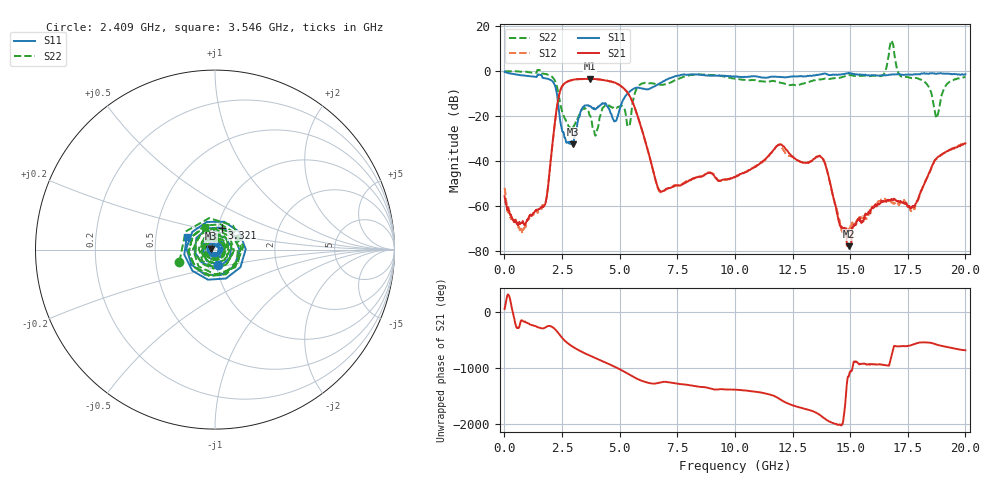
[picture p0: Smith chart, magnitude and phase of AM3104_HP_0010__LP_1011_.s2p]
!Created with skrf (http://scikit-rf.org).
# Hz S RI R 50.0
!freq ReS11 ImS11 ReS21 ImS21 ReS12 ImS12 ReS22 ImS22
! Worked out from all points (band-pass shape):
!   1601 points, 10 MHz to 20 GHz, reference 50 ohm
!   highest |S21| = -3.39 dB at 3.708 GHz (marker M1); lowest = -77.8 dB at 14.95 GHz (marker M2)
!   |S21| within 3 dB of the highest: 2.526 GHz to 5.028 GHz (2.502 GHz wide, 66.3 % of centre)
!   lowest |S11| = -32.5 dB at 2.984 GHz (marker M3), VSWR 1.05, Z = 47.7 + j0.478 ohm
!   |S11| at or under -10 dB: 2.276 GHz to 5.339 GHz (3.063 GHz wide, 80.4 % of centre)
!   |S22| runs from -28.7 to 13.6 dB; largest |S21 - S12| = 0.055
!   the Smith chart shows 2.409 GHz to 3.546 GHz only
!   S11 on the Smith chart (normalised r, x): 2.409 GHz: 1.02, -0.18; 3.321 GHz: 1.05, +0.26; 3.546 GHz: 0.72, +0.11
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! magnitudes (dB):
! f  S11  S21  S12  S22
! 10 MHz  -0.3  -55.6  -51.9  -0.1
! 722.1 MHz  -1.9  -67.5  -70.1  -0.3
! 1.697 GHz  -3.1  -60.4  -59.7  -1.1
! 2.409 GHz  -21.1  -9.1  -9.2  -13.6
! 2.984 GHz  -32.5  -3.8  -3.8  -24.8
! 3.321 GHz  -17.8  -3.5  -3.6  -17.9
! 3.346 GHz  -17.2  -3.5  -3.6  -17.2
! 3.546 GHz  -15.2  -3.4  -3.5  -17.1
! 3.708 GHz  -15.6  -3.4  -3.5  -19.8
! 4.808 GHz  -22.2  -5.1  -5.2  -16.5
! 5.395 GHz  -9.5  -10.3  -10.4  -24.6
! 5.807 GHz  -7.3  -20.8  -20.8  -6.8
! 6.682 GHz  -5.8  -52.3  -52.5  -5.9
! 10.01 GHz  -2.5  -47.1  -47.1  -3.4
! 11.93 GHz  -2.6  -32.5  -32.8  -5.0
! 13.34 GHz  -2.1  -39.8  -39.9  -4.4
! 13.87 GHz  -1.1  -40.1  -39.7  -3.4
! 14.95 GHz  -0.8  -77.8  -70.0  -1.8
! 16.68 GHz  -1.6  -57.5  -57.8  7.3
! 17.71 GHz  -1.5  -60.2  -61.7  -3.1
! 18.75 GHz  -1.2  -38.8  -38.9  -20.9
! 20 GHz  -1.4  -32.1  -31.8  -2.7
